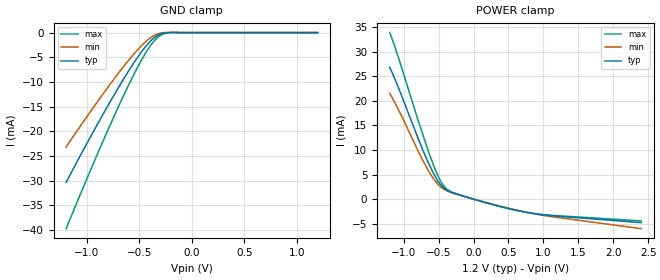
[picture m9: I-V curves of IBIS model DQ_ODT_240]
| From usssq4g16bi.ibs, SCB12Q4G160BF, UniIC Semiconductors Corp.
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|   Model DQ_ODT_240
[Model] DQ_ODT_240
Model_type Input
Polarity   Non-Inverting
Enable   Active-High
Vinl =  8.300E-01
Vinh =  9.700E-01
C_comp   8.371E-13   8.307E-13   8.473E-13
C_comp_power_clamp   2.926E-13   2.899E-13   2.983E-13
C_comp_gnd_clamp   5.445E-13   5.408E-13   5.490E-13
[Model Spec]
Vinh   9.700E-01   9.250E-01   1.015E+00
Vinl   8.300E-01   7.850E-01   8.750E-01
[Temperature Range]   45.000   95.000   -40.000
[Voltage Range]   1.200E+00   1.140E+00   1.260E+00
[C Comp Corner]
C_comp_power_clamp   2.926E-13   2.983E-13   2.899E-13
C_comp_gnd_clamp   5.445E-13   5.490E-13   5.408E-13
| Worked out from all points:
|   GND clamp passes 1 mA (typ) near -0.36 V on its own axis
|   POWER clamp passes 1 mA (typ) near -0.24 V on its own axis
[GND_clamp]
|Voltage   I(typ)   I(min)   I(max)
-1.2V     -30.32mA   -23.17mA   -39.72mA
-875mV    -17.58mA   -13.23mA   -23.31mA
-750mV    -12.92mA   -9.601mA   -17.3mA
-625mV    -8.493mA   -6.167mA   -11.58mA
-525mV    -5.226mA   -3.657mA   -7.316mA
-450mV    -3.055mA   -2.021mA   -4.444mA
-375mV    -1.316mA   -767uA     -2.068mA
-325mV    -542.1uA   -255.6uA   -937.8uA
-275mV    -140.9uA   -20.17uA   -291.3uA
-200mV    9.625uA    43.66uA    -13.12uA
1.2V      0A         0A         0A
[POWER_clamp]
|Voltage   I(typ)   I(min)   I(max)
-1.2V     26.82mA    21.52mA    33.92mA
-1.075V   22.69mA    18.23mA    28.79mA
-750mV    10.85mA    8.579mA    14.15mA
-600mV    6.007mA    4.74mA     7.941mA
-475mV    3.005mA    2.546mA    3.783mA
-425mV    2.255mA    2.008mA    2.664mA
-375mV    1.759mA    1.629mA    1.941mA
-250mV    1.058mA    1.006mA    1.108mA
200mV     -804.8uA   -771.1uA   -838.1uA
800mV     -2.786mA   -2.804mA   -2.794mA
1.125V    -3.396mA   -3.587mA   -3.312mA
2.4V      -4.788mA   -6.015mA   -4.439mA
